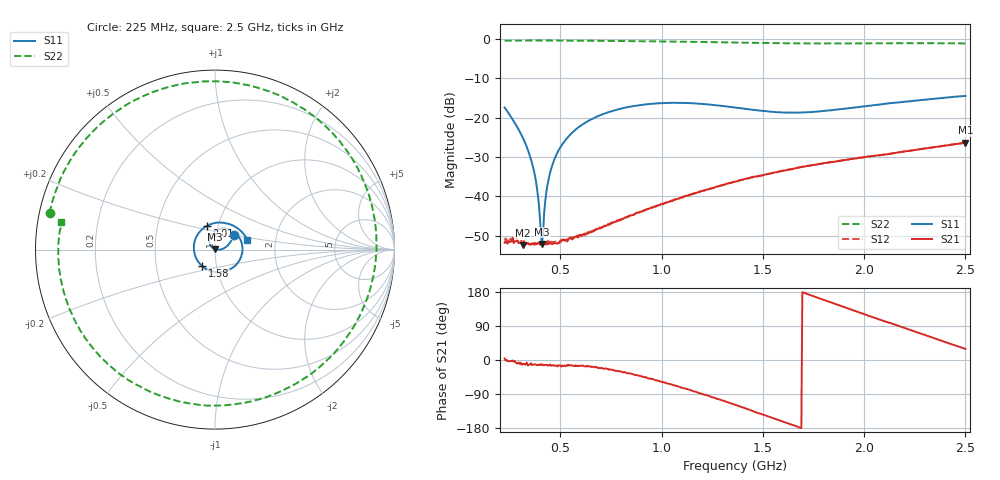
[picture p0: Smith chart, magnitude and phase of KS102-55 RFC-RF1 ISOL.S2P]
!Agilent	"Technologies,E8364B,MY43040668,A.07.50.67"
!Agilent	E8364B:	A.07.50.67
!Date:	"Tuesday,"	September	"22,"	2015	13:37:09
!Correction:	S11(Full	2	"Port(1,2))"
!S21(Full	2	"Port(1,2))"
!S12(Full	2	"Port(1,2))"
!S22(Full	2	"Port(1,2))"
!S2P	File:	Measurements:	"S11,"	"S21,"	"S12,"	S22:
#	Hz	S	dB	R	50
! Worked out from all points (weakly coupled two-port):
!   456 points, 225 MHz to 2.5 GHz, reference 50 ohm
!   highest |S21| = -26.34 dB at 2.5 GHz (marker M1); lowest = -52.3 dB at 315 MHz (marker M2)
!   lowest |S11| = -52.0 dB at 410 MHz (marker M3), VSWR 1.01, Z = 50 + j0.25 ohm
!   |S11| at or under -10 dB: start of sweep to end of sweep
!   |S22| runs from -1.2 to -0.5 dB; largest |S21 - S12| = 0.00046
!   S11 on the Smith chart (normalised r, x): 225 MHz: 1.21, +0.21; 1.58 GHz: 0.85, -0.16; 2.01 GHz: 0.88, +0.24; 2.5 GHz: 1.43, +0.16
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2.25e8  -17.47 38.7  -51.72 4.2  -51.17 0.1  -0.50 167.5
3.15e8  -25.18 10.6  -52.35 -11.0  -51.79 -8.9  -0.47 148.5
3.7e8  -33.52 -1.5  -51.84 -11.5  -52.62 -12.8  -0.48 138.7
3.85e8  -38.05 -4.1  -52.00 -13.6  -51.87 -14.1  -0.47 136.0
4.05e8  -50.21 30.0  -52.11 -13.6  -51.74 -15.1  -0.48 132.7
4.1e8  -52.04 89.9  -51.66 -11.0  -52.31 -16.7  -0.48 131.8
4.15e8  -49.42 125.5  -51.84 -13.8  -52.47 -17.3  -0.48 131.0
4.4e8  -36.19 143.2  -52.19 -15.1  -51.31 -14.1  -0.48 126.9
4.7e8  -30.67 139.5  -51.59 -15.4  -51.60 -15.4  -0.48 122.0
5.25e8  -25.75 126.9  -51.09 -16.4  -51.25 -13.1  -0.51 113.3
6.05e8  -21.91 108.3  -50.04 -15.2  -50.01 -16.1  -0.53 101.2
7.95e8  -17.80 64.5  -46.04 -29.9  -45.84 -30.5  -0.61 73.4
9.85e8  -16.39 23.7  -42.19 -54.8  -42.31 -55.5  -0.71 46.2
1.185e9  -16.49 -20.3  -38.92 -87.3  -38.83 -87.3  -0.84 16.3
1.365e9  -17.49 -64.8  -36.23 -118.3  -36.19 -118.2  -0.99 -12.4
1.58e9  -18.65 -128.0  -33.68 -158.8  -33.71 -158.9  -1.15 -49.2
1.745e9  -18.60 -179.8  -32.04 169.3  -32.06 169.2  -1.23 -77.8
1.865e9  -18.00 145.4  -31.10 146.5  -31.08 146.8  -1.23 -97.8
2.01e9  -17.12 108.8  -29.98 119.1  -29.95 119.3  -1.20 -121.0
2.125e9  -16.39 83.8  -29.21 98.3  -29.21 98.4  -1.17 -138.1
2.315e9  -15.41 48.6  -27.77 63.3  -27.73 63.6  -1.16 -164.8
2.5e9  -14.54 17.1  -26.34 29.3  -26.31 29.4  -1.21 169.8
